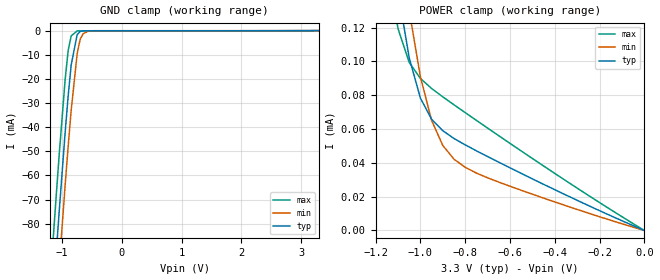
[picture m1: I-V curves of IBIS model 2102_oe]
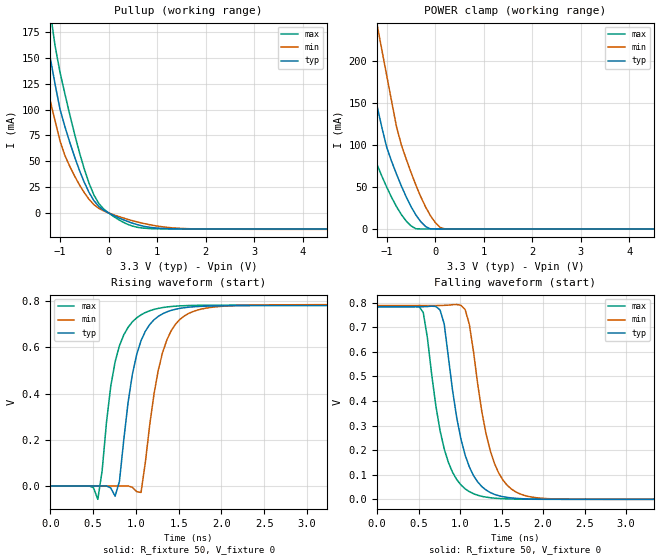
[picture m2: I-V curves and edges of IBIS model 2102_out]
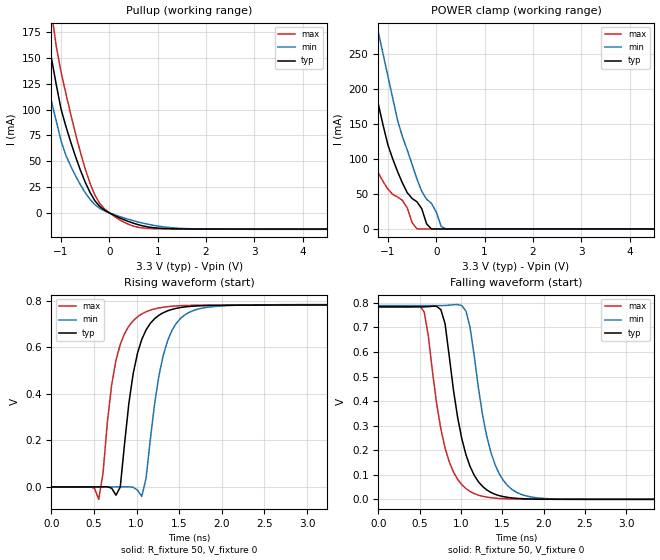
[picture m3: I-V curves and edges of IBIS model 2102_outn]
| IBIS File eg2102h.ibs
[IBIS ver]   3.2
[File name]   eg2102h.ibs
[File Rev]   1.0
[Date]   July 8,2010
[Source]   Circiuts Simulation for EG-2102CA HCSL by HSPICE
|   Component EG-2102CA HCSL
[Component]   EG-2102H
[Manufacturer]   Epson Toyocom Corp.
[Package]
| variable   typ   min   max
R_pkg   1.04   NA   NA
L_pkg   1.98n   NA   NA
C_pkg   3.71p   NA   NA
[Pin]   signal_name   model_name   R_pin   L_pin   C_pin
1   oe   2102_oe   NA   NA   NA
|2   nc   dummy
3   vss   GND   NA   NA   NA
4   out   2102_out   1.04   1.98n   3.71p
5   outn   2102_outn   1.04   1.98n   3.71p
6   vdd   POWER   NA   NA   NA
[Diff Pin] inv_pin vdiff   tdelay_typ
4   5   0.4   0
| Models and submodels in the file (3): 2102_oe (Input), 2102_out (Open_source), 2102_outn (Open_source)
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|   Model 2102_oe
[Model]   2102_oe
Model_type   Input
Vinh   = 2.31V
Vinl   = 0.99V
C_comp   3pF   NA   NA
|   typ   min   max
[Temperature Range]   25.00  -40.00   85.00
[Voltage Range]   3.30V   3.00V   3.60V
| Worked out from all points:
|   GND clamp passes 1 mA (typ) near -0.72 V on its own axis
|   POWER clamp passes 1 mA (typ) near -1.64 V on its own axis
[GND_clamp]
|voltage   current   current   current
|vout   I(typ)   I(min)   I(max)
-3.3V     -919.3mA   -939.8mA   -898.4mA
-1.15V    -109.5mA   -132.2mA   -85.74mA
-1.1V     -91.92mA   -114.6mA   -68.2mA
-1.05V    -74.68mA   -97.25mA   -51.14mA
-950mV    -41.84mA   -63.68mA   -19.99mA
-900mV    -26.97mA   -47.81mA   -8.167mA
-850mV    -14.25mA   -32.98mA   -2.19mA
-750mV    -1.706mA   -9.619mA   -128.9uA
-700mV    -343.6uA   -3.593mA   -111.9uA
-650mV    -108.1uA   -1.289mA   -110.4uA
-550mV    -69.46uA   -93.35uA   -110.2uA
3.3V      3.304pA    12.42uA    -22.73uA
[POWER_clamp]
|vout   I(typ)   I(min)   I(max)
-3.3V     4.199mA    4.231mA    4.175mA
-1.1V     141.6uA    182uA      119.5uA
-1.05V    102.2uA    130.2uA    99.43uA
-1V       78.31uA    90.94uA    89.93uA
-950mV    65.8uA     65.14uA    83.99uA
-900mV    58.99uA    50.29uA    79.04uA
-850mV    54.42uA    42.17uA    74.34uA
-800mV    50.63uA    37.35uA    69.72uA
-750mV    47.13uA    33.96uA    65.13uA
-650mV    40.38uA    28.61uA    56.04uA
-300mV    17.83uA    12.42uA    25.04uA
0V        3.297pA    3.975pA    3.602pA
|   Model 2102_out
[Model]   2102_out
Model_type   Open_source
Polarity   Non-Inverting
Enable   Active-High
Vref   = 0
Vmeas   = 0.4
Rref   = 50.0
C_comp   3pF   NA   NA
|   typ   min   max
[Temperature Range]   25.00  -40.00   85.00
[Voltage Range]   3.30V   3.00V   3.60V
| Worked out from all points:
|   slope of the pullup table from 0 to 0.495 V, typ, clamps not added: 49.6 ohm
|   POWER clamp passes 1 mA (typ) near -0.13 V on its own axis
|   falling waveform, R_fixture 50, V_fixture 0: 20-80 % time 244ps typ, 255ps min, 236ps max; typ from 0.783 V to 0 V
|   rising waveform, R_fixture 50, V_fixture 0: 20-80 % time 211ps typ, 231ps min, 202ps max; typ from 0 V to 0.781 V
[POWER_clamp]
|vout   I(typ)   I(min)   I(max)
-3.3V     705mA      874.5mA    562mA
-2V       359.6mA    491.4mA    253.8mA
-1.9V     332.6mA    460.6mA    230.5mA
-1.6V     251.8mA    368mA      161.6mA
-1.5V     225.1mA    336.8mA    139mA
-1.2V     146.2mA    243.6mA    76.66mA
-1V       96.87mA    182.2mA    49.56mA
-800mV    65.34mA    121.7mA    26.53mA
-400mV    16.56mA    52.08mA    242.5uA
-100mV    28.71uA    15.67mA    -457.1nA
200mV     -4.919nA   198.6nA    -489.5nA
6.6V      -8.183nA   -958.4pA   -688.6nA
[Pullup]
|vout   I(typ)   I(min)   I(max)
-3.3V     701mA      531.8mA    891.8mA
-1.6V     254.5mA    186.6mA    329.7mA
-1.5V     228.1mA    166.9mA    295.6mA
-1.3V     175.9mA    127.8mA    228.2mA
-1.2V     150mA      108.3mA    194.7mA
-1V       100.4mA    69.68mA    136.2mA
-900mV    83.68mA    55.68mA    115.5mA
-400mV    19.68mA    13.07mA    28.54mA
-100mV    2.63mA     1.897mA    3.796mA
400mV     -8.411mA   -6.323mA   -11.18mA
1.6V      -15.59mA   -15.26mA   -15.6mA
6.6V      -15.79mA   -16.17mA   -15.75mA
[Falling Waveform]
R_fixture   = 50
V_fixture   = 0
0s        783.5mV    788.7mV    783.9mV
555.6ps   783.9mV    788.7mV    760.2mV
757.6ps   771mV      789mV      280.5mV
808.1ps   713.8mV    789.5mV    205.4mV
909.1ps   442.2mV    792.1mV    109.8mV
1.061ns   179.8mV    772.1mV    42.75mV
1.162ns   96.48mV    599.6mV    22.77mV
1.364ns   27.55mV    197.1mV    6.469mV
1.717ns   3.049mV    22.64mV    746.6uV
5ns       1.236uV    8.513uV    1.363uV
[Rising Waveform]
R_fixture   = 50
V_fixture   = 0
0s        0V         0V         0V
555.6ps   121.2uV    -13.2uV    -57.61mV
757.6ps   -43.81mV   86.25uV    537.1mV
808.1ps   19.83mV    235.8uV    606.5mV
959.6ps   483.3mV    -5.637mV   710.1mV
1.061ns   628.6mV    -27.76mV   740.5mV
1.111ns   669.6mV    102.6mV    750.4mV
1.313ns   745mV      578.4mV    771.8mV
1.616ns   773.4mV    746.3mV    780.6mV
5ns       780.9mV    785.1mV    783.5mV
[Ramp]
R_load   = 50
dV/dt_r   4.685E-1/2.100E-10   4.711E-1/2.304E-10   4.701E-1/2.005E-10
dV/dt_f   4.701E-1/2.410E-10   4.732E-1/2.518E-10   4.703E-1/2.358E-10
| End [Model] 2102_out
|   Model 2102_outn
[Model]   2102_outn
Model_type   Open_source
Polarity   Non-Inverting
Enable   Active-High
Vref   = 0
Vmeas   = 0.4
Rref   = 50.0
C_comp   3pF   NA   NA
|   typ   min   max
[Temperature Range]   25.00  -40.00   85.00
[Voltage Range]   3.30V   3.00V   3.60V
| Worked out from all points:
|   slope of the pullup table from 0 to 0.495 V, typ, clamps not added: 49.6 ohm
|   POWER clamp passes 1 mA (typ) near -0.11 V on its own axis
|   falling waveform, R_fixture 50, V_fixture 0: 20-80 % time 245ps typ, 256ps min, 236ps max; typ from 0.783 V to 0 V
|   rising waveform, R_fixture 50, V_fixture 0: 20-80 % time 203ps typ, 216ps min, 194ps max; typ from 0 V to 0.782 V
[POWER_clamp]
|vout   I(typ)   I(min)   I(max)
-3.3V     796.8mA    887.5mA    576.4mA
-2.1V     446.7mA    564.8mA    280.2mA
-1.6V     298.8mA    408mA      162.9mA
-1.5V     269.1mA    376.2mA    140.2mA
-1.2V     178.3mA    280.9mA    79.97mA
-1V       119.7mA    217.5mA    56.69mA
-800mV    81.68mA    154.6mA    45.48mA
-600mV    51.59mA    112.4mA    30.04mA
-400mV    38.75mA    71.21mA    198.7uA
-100mV    17.93uA    36.54mA    780.7pA
200mV     5.142pA    123.8nA    -908.2fA
6.6V      -10.43pA   -10.17pA   -13.74pA
[Pullup]
|vout   I(typ)   I(min)   I(max)
-3.3V     701mA      531.8mA    891.8mA
-1.6V     254.5mA    186.6mA    329.7mA
-1.5V     228.1mA    166.9mA    295.6mA
-1.3V     175.9mA    127.8mA    228.2mA
-1.2V     150mA      108.3mA    194.7mA
-1V       100.4mA    69.68mA    136.2mA
-900mV    83.68mA    55.68mA    115.5mA
-400mV    19.68mA    13.07mA    28.54mA
-100mV    2.63mA     1.897mA    3.796mA
400mV     -8.411mA   -6.323mA   -11.18mA
1.6V      -15.59mA   -15.26mA   -15.6mA
6.6V      -15.79mA   -16.17mA   -15.75mA
[Falling Waveform]
R_fixture   = 50
V_fixture   = 0
0s        783.5mV    788.7mV    783.9mV
555.6ps   783.5mV    788.7mV    762.8mV
757.6ps   771.9mV    788.6mV    285.7mV
808.1ps   715.1mV    789.2mV    209.3mV
909.1ps   446.5mV    792.2mV    111.8mV
1.061ns   182mV      766.7mV    43.59mV
1.162ns   97.68mV    582.5mV    23.22mV
1.364ns   27.88mV    190.2mV    6.598mV
1.717ns   3.097mV    21.83mV    750uV
5ns       7.96uV     -2.866uV   3.412uV
[Rising Waveform]
R_fixture   = 50
V_fixture   = 0
0s        0V         0V         0V
555.6ps   44.98uV    4.809uV    -53.32mV
757.6ps   -35.41mV   580.8nV    543.9mV
808.1ps   -234uV     117.6uV    612.6mV
959.6ps   486.8mV    -1.684mV   714mV
1.061ns   633.9mV    -40.95mV   743.2mV
1.111ns   674.7mV    38.47mV    752.5mV
1.313ns   748.5mV    566.4mV    772mV
1.616ns   775.2mV    749.8mV    779.8mV
5ns       782.4mV    783.6mV    782.5mV
[Ramp]
R_load   = 50
dV/dt_r   4.695E-1/2.017E-10   4.702E-1/2.155E-10   4.695E-1/1.933E-10
dV/dt_f   4.701E-1/2.416E-10   4.732E-1/2.526E-10   4.703E-1/2.362E-10
| End [Model] 2102_outn
| End [Component] EG-2102H
